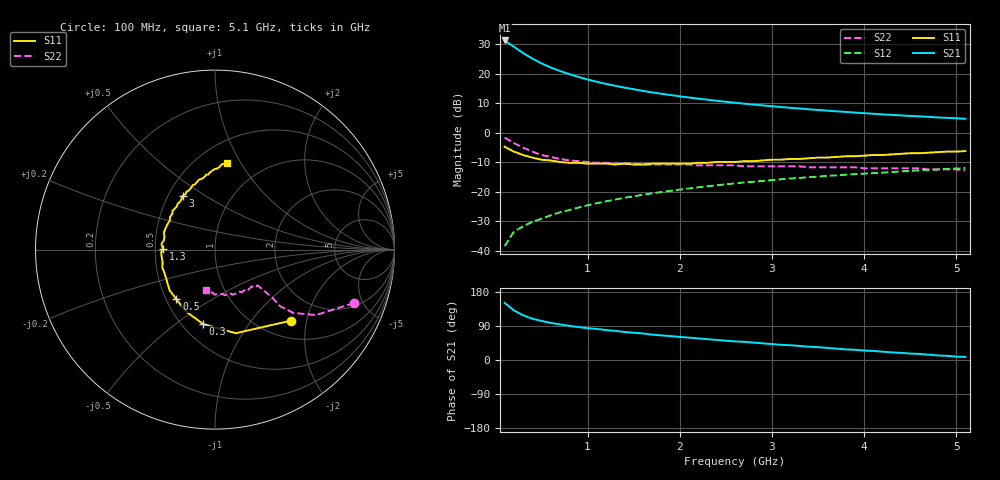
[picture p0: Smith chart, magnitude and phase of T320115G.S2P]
!AT-32011
!S and NOISE PARAMETERS at Vce=5  V  Ic=20mA.  LAST UPDATED 01-05-95
# ghz s ma r 50
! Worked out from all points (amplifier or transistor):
!   51 points, 100 MHz to 5.1 GHz, reference 50 ohm
!   highest |S21| = 31.3 dB at 100 MHz (marker M1)
!   |S21| within 3 dB of that: start of sweep to 241 MHz
!   unconditionally stable (mu >= 1): 976.8 MHz to 4.781 GHz
!   at 900 MHz: K = 0.98, MSG = 22.1 dB, |S12| = -25.4 dB
!   at 2.6 GHz: K = 1.07, MAG = 12.1 dB, |S12| = -17.1 dB
!   at 5.1 GHz: K = 0.99, MSG = 8.4 dB, |S12| = -12.0 dB
!   lowest NFmin = 1.38 dB at 500 MHz
!   S11 on the Smith chart (normalised r, x): 100 MHz: 1.36, -1.62; 300 MHz: 0.63, -0.63; 500 MHz: 0.56, -0.36; 1.3 GHz: 0.55, +0.01; 3 GHz: 0.59, +0.40; 5.1 GHz: 0.69, +0.88
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0.1  0.58 -43.0  36.64 151.0  0.012 72.0  0.83 -21.0
0.2  0.48 -76.0  28.69 131.0  0.021 64.0  0.67 -33.0
0.3  0.42 -99.0  22.44 118.0  0.026 61.0  0.56 -39.0
0.4  0.38 -116.0  18.09 109.0  0.031 61.0  0.48 -41.0
0.5  0.35 -128.0  14.99 103.0  0.035 62.0  0.42 -40.0
0.6  0.34 -138.0  12.79 98.0  0.04 63.0  0.39 -40.0
0.7  0.32 -147.0  11.14 94.0  0.045 63.0  0.36 -40.0
0.8  0.31 -155.0  9.86 90.0  0.049 64.0  0.34 -40.0
0.9  0.31 -161.0  8.84 87.0  0.054 64.0  0.33 -40.0
1  0.3 -167.0  8 84.0  0.059 64.0  0.32 -40.0
1.2  0.3 -177.0  6.74 79.0  0.069 64.0  0.31 -41.0
1.3  0.29 179.0  6.25 77.0  0.074 63.0  0.3 -42.0
1.4  0.3 174.0  5.83 74.0  0.079 63.0  0.3 -43.0
1.5  0.29 170.0  5.46 72.0  0.084 63.0  0.3 -44.0
1.8  0.3 158.0  4.58 65.0  0.099 61.0  0.29 -47.0
2.2  0.31 144.0  3.79 57.0  0.119 58.0  0.28 -52.0
2.6  0.32 132.0  3.23 49.0  0.139 55.0  0.28 -58.0
3  0.35 121.0  2.82 42.0  0.158 52.0  0.27 -64.0
3.5  0.38 109.0  2.44 34.0  0.181 47.0  0.26 -72.0
3.8  0.4 103.0  2.26 28.0  0.195 44.0  0.26 -76.0
4.3  0.43 94.0  2.01 20.0  0.216 40.0  0.25 -84.0
5.1  0.49 82.0  1.73 8.0  0.252 32.0  0.23 -102.0
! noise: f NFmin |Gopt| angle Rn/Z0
0.5  1.38  0.18  50  0.2
0.9  1.5  0.15  88  0.16
1.8  1.78  0.23  176  0.13
2.4  1.96  0.34  -156  0.12
